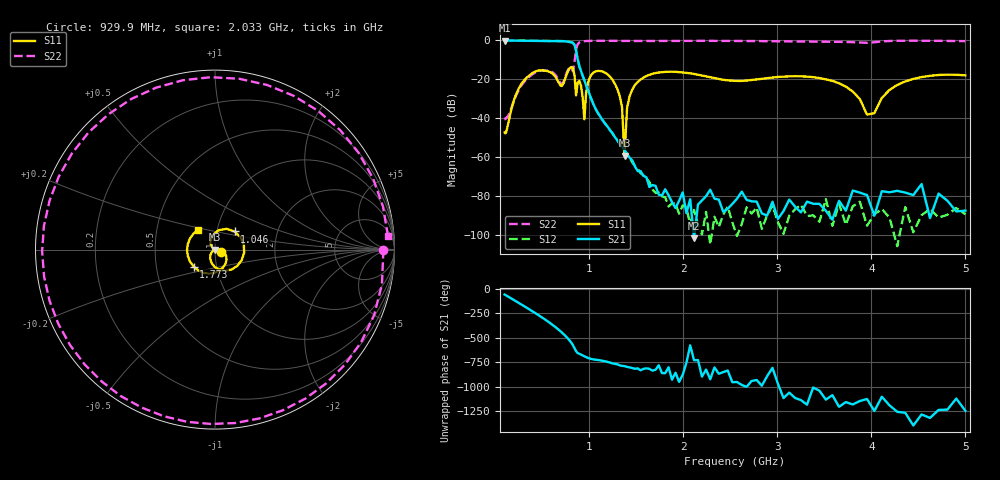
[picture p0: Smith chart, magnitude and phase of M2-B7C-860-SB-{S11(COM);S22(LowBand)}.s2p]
!Agilent Technologies,N5230A,MY45001737,A.07.50.48
!Agilent N5230A: A.07.50.48
!Date: Friday, August 11, 2023 17:37:03
!Correction: S11(Full 2 Port(1,4))
!S41(Full 2 Port(1,4))
!S14(Full 2 Port(1,4))
!S44(Full 2 Port(1,4))
!S2P File: Measurements: S11, S41, S14, S44:Log Frequency Sweep
# Hz S  MA  R 50
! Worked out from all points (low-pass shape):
!   201 points, 100 MHz to 5 GHz, reference 50 ohm
!   highest |S21| = -0.10 dB at 106 MHz (marker M1); lowest = -101.8 dB at 2.114 GHz (marker M2)
!   |S21| within 3 dB of the highest: start of sweep to 847.6 MHz
!   lowest |S11| = -59.3 dB at 1.375 GHz (marker M3), VSWR 1.00, Z = 50 - j0.104 ohm
!   |S11| at or under -10 dB: start of sweep to end of sweep
!   |S22| runs from -40.6 to -0.2 dB; largest |S21 - S12| = 0.0046
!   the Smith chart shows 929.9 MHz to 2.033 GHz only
!   S11 on the Smith chart (normalised r, x): 929.9 MHz: 1.06, -0.03; 1.046 GHz: 1.22, +0.25; 1.773 GHz: 0.78, -0.15; 2.033 GHz: 0.81, +0.18
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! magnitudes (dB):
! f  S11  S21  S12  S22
! 100 MHz  -47.3  -0.1  -0.1  -40.5
! 106 MHz  -47.7  -0.1  -0.1  -40.6
! 425.2 MHz  -16.1  -0.3  -0.3  -16.6
! 707.1 MHz  -23.5  -0.4  -0.4  -22.4
! 810.9 MHz  -13.7  -1.1  -1.0  -14.2
! 929.9 MHz  -29.3  -18.2  -18.2  -0.6
! 948.2 MHz  -40.6  -20.6  -20.6  -0.4
! 1.046 GHz  -16.6  -33.0  -33.0  -0.3
! 1.297 GHz  -24.7  -51.3  -51.2  -0.3
! 1.348 GHz  -34.2  -54.7  -54.8  -0.3
! 1.375 GHz  -59.3  -56.4  -56.7  -0.3
! 1.402 GHz  -34.8  -58.5  -58.5  -0.3
! 1.458 GHz  -25.2  -61.8  -62.7  -0.3
! 1.739 GHz  -16.6  -79.3  -78.1  -0.3
! 1.773 GHz  -16.4  -79.8  -80.2  -0.3
! 2.033 GHz  -16.7  -88.8  -86.1  -0.3
! 2.114 GHz  -17.3  -101.8  -87.2  -0.3
! 2.571 GHz  -20.9  -81.4  -100.5  -0.3
! 3.381 GHz  -18.9  -84.0  -89.9  -0.7
! 3.954 GHz  -38.2  -79.6  -95.3  -1.3
! 4.193 GHz  -25.5  -78.1  -91.1  -0.3
! 5 GHz  -18.0  -87.5  -89.4  -0.4
